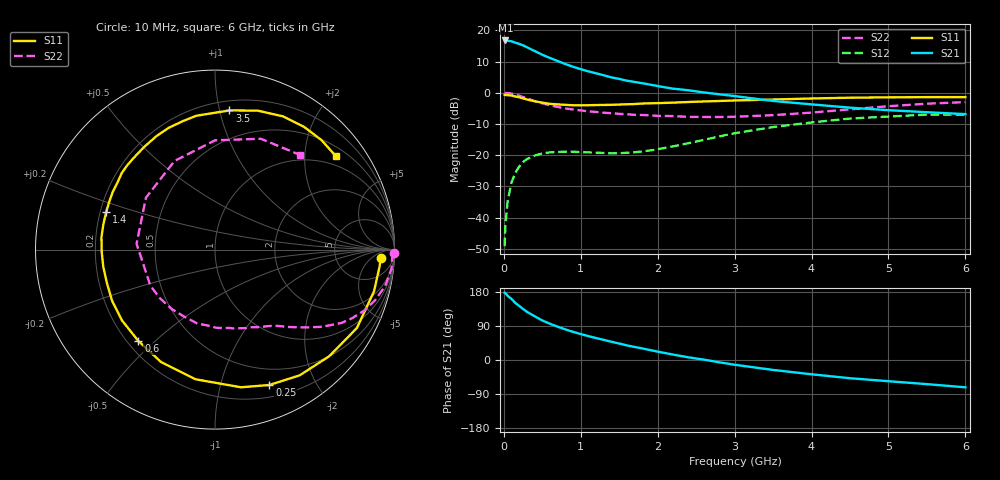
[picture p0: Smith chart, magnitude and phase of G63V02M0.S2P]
! SIEMENS Small Signal Semiconductors
! BFG193
! Si NPN RF Bipolar Junction Transistor in SOT223
! VCE = 3 V  IC = 2 mA
! Common Emitter S-Parameters:  August  1996
# GHz  S  MA  R  50
!  f  S11  S21  S12  S22
! GHz  MAG  ANG  MAG  ANG  MAG  ANG  MAG  ANG
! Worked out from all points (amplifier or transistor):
!   36 points, 10 MHz to 6 GHz, reference 50 ohm
!   highest |S21| = 16.7 dB at 20 MHz (marker M1)
!   |S21| within 3 dB of that: start of sweep to 368.9 MHz
!   unconditionally stable (mu >= 1): 1.359 GHz to 2.58 GHz
!   at 250 MHz: K = 0.18, MSG = 18.7 dB, |S12| = -22.2 dB
!   at 1.4 GHz: K = 1.04, MAG = 11.0 dB, |S12| = -19.4 dB
!   at 6 GHz: K = 0.96, MSG = 0.1 dB, |S12| = -7.0 dB
!   S11 on the Smith chart (normalised r, x): 10 MHz: 18, -12; 250 MHz: 0.32, -1.43; 600 MHz: 0.24, -0.44; 1.4 GHz: 0.22, +0.16; 3.5 GHz: 0.27, +1.07; 6 GHz: 0.73, +2.76
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0.01  0.9246 -2.9  6.846 177.8  0.0035 90.8  0.9962 -1.2
0.02  0.9219 -5.9  6.876 176.7  0.0075 89.7  0.9885 -2.4
0.05  0.9159 -14.7  6.801 169.2  0.0185 81.1  0.989 -6.2
0.1  0.9034 -28.9  6.659 161.0  0.0366 74.3  0.9695 -12.1
0.15  0.8707 -43.0  6.329 150.4  0.0526 66.0  0.9351 -17.6
0.25  0.8129 -68.1  5.737 134.4  0.078 53.4  0.854 -26.6
0.3  0.7807 -79.3  5.354 127.2  0.0866 48.3  0.8148 -30.1
0.4  0.7306 -98.6  4.663 115.5  0.0987 39.5  0.7367 -35.7
0.5  0.695 -115.6  4.056 104.3  0.1069 32.4  0.677 -39.8
0.6  0.6645 -130.0  3.608 95.6  0.1112 27.7  0.6299 -43.4
0.7  0.6514 -142.6  3.222 87.8  0.1128 23.8  0.5931 -46.6
0.8  0.6406 -153.4  2.88 80.8  0.1139 20.8  0.5618 -49.4
0.9  0.6305 -162.7  2.607 74.3  0.1137 19.2  0.5391 -51.9
1.1  0.6315 -178.9  2.201 62.9  0.1109 17.4  0.5046 -58.3
1.4  0.6412 161.0  1.76 48.1  0.1072 18.7  0.4704 -68.4
1.6  0.6543 150.3  1.559 38.5  0.1096 22.0  0.4528 -76.2
2.2  0.695 124.6  1.164 14.3  0.1386 31.4  0.4229 -103.6
2.8  0.7379 104.0  0.946 -6.1  0.2002 29.7  0.4092 -138.2
3.5  0.7795 84.1  0.739 -26.2  0.2826 15.5  0.4381 175.8
4.5  0.8334 63.0  0.577 -48.1  0.3866 -8.7  0.5427 114.6
5.5  0.851 45.8  0.488 -63.7  0.4469 -37.2  0.6684 67.5
6  0.8512 37.6  0.455 -72.1  0.4483 -52.6  0.7087 48.1
